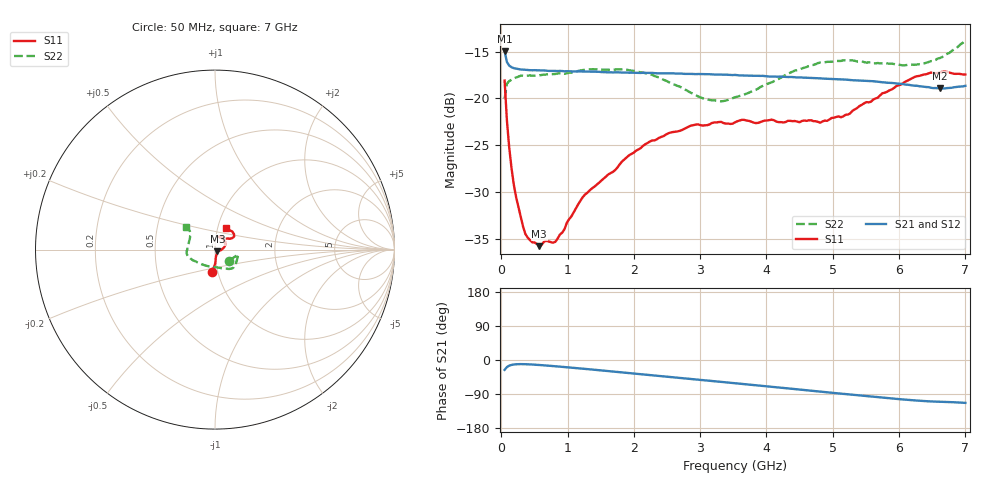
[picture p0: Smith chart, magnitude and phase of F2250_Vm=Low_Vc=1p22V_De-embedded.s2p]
! Integrated Device Technology
! Corporate Headquarters
! 6024 Silver Creek Valley Road
! San Jose, CA 95138  USA
! Phone:  1-408-284-8200
! Toll Free:  1-800-223-1366
! Webpage:  http://www.idt.com/
! Timing and RF Division
! 515 Groton Road, Suite 102
! Westford, MA 01886-6024
! Device:  F2250
! Description: Voltage Variable RF Attenuator
! Frequency:  50.0 -  6000.00 MHz
! Package:  3x3 mm Thin QFN Plastic Package: 16 pin
! Ports:  2 RF, 3 DC
!  Pin  1  = GND
!  Pin  2  = NC
!  Pin  3  = RF1  = Port 1
!  Pin  4  = NC
!  Pin  5  = GND
!  Pin  6  = GND
!  Pin  7  = GND
!  Pin  8  = GND
!  Pin  9  = NC
!  Pin 10  = RF2  = Port 2
!  Pin 11  = NC
!  Pin 12  = GND
!  Pin 13  = GND
!  Pin 14  = VCNTRL
!  Pin 15  = VDD
!  Pin 16  = VMODE
! Vcntrl:  1.220 Volts
! Vmode:  +0.000 Volts
! Vdd:  +3.30  Volts
! Current:  1.195 mA
! Data:  The device was measured on a the F2250 evaluation board which has
!  individual transmission lines to the RF pins.  Data was collected
!  using a calibrated network analyzer.  The evaluation board was
!  de-embedded using a TRL calibration technique.
!  The reference plane is the edge of the package pin.
! Misc:  SN 10
!  Action Tracker AT0258
! Date Measured:  2014-11-26
! Date:  2015-10-15  MJV
! Note:
!  Integrated Device Technology supplies this data as a sample of measured
!  data at the package pin for this product.  Your particular data for this
!  product may vary.
!  Data was taken at 25 degrees C.
!  Integrated Device Technology reserves the right to change this data at anytime.
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# GHz S dB R 50
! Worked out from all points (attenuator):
!   201 points, 50 MHz to 7 GHz, reference 50 ohm
!   highest |S21| = -14.97 dB at 50 MHz (marker M1); lowest = -18.9 dB at 6.618 GHz (marker M2)
!   lowest |S11| = -35.8 dB at 571.2 MHz (marker M3), VSWR 1.03, Z = 51.4 - j0.895 ohm
!   |S11| at or under -10 dB: start of sweep to end of sweep
!   |S22| runs from -20.3 to -13.8 dB; largest |S21 - S12| = 0.00051
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0.05  -18.09 -97.1  -14.97 -25.9  -14.96 -25.9  -20.04 -37.6
0.08475  -22.36 -88.8  -16.10 -18.6  -16.09 -18.6  -18.44 -18.3
0.1195  -25.26 -86.0  -16.49 -14.9  -16.49 -14.9  -18.15 -13.4
0.15425  -27.47 -83.6  -16.67 -13.0  -16.67 -12.9  -18.01 -12.0
0.22375  -30.58 -73.2  -16.81 -11.2  -16.81 -11.2  -17.77 -12.0
0.36275  -34.51 -57.2  -16.94 -11.1  -16.95 -11.1  -17.57 -13.1
0.57125  -35.82 -32.5  -17.00 -13.1  -17.00 -13.1  -17.53 -18.3
0.6755  -35.25 -29.5  -17.03 -14.5  -17.04 -14.5  -17.44 -21.0
0.8145  -35.36 -19.4  -17.06 -16.5  -17.06 -16.5  -17.38 -25.1
1.2315  -30.54 -8.1  -17.13 -22.9  -17.14 -22.9  -16.96 -35.1
1.9265  -26.09 12.3  -17.26 -34.2  -17.26 -34.2  -16.98 -47.1
2.37825  -24.22 23.7  -17.31 -41.7  -17.31 -41.7  -17.75 -56.3
2.86475  -22.91 39.1  -17.38 -50.0  -17.40 -50.0  -19.41 -73.7
3.0385  -22.91 45.6  -17.40 -53.0  -17.41 -53.0  -19.99 -83.1
3.3165  -22.52 54.7  -17.46 -57.7  -17.47 -57.7  -20.31 -101.6
3.525  -22.56 59.7  -17.49 -61.3  -17.51 -61.3  -19.88 -115.6
4.7065  -22.43 66.3  -17.82 -81.6  -17.82 -81.6  -16.42 -163.0
5.22775  -21.73 49.2  -18.01 -90.5  -18.02 -90.5  -15.94 -173.0
5.85325  -19.14 34.3  -18.33 -100.9  -18.33 -101.0  -16.29 173.0
6.2355  -17.70 34.9  -18.65 -106.5  -18.63 -106.6  -16.40 160.0
6.61775  -17.21 43.4  -18.94 -110.1  -18.93 -110.1  -15.68 146.6
7  -17.44 63.2  -18.65 -113.2  -18.63 -113.3  -13.80 142.4
